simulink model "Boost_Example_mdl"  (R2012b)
settings: Solver=ode45  StartTime=0.0  StopTime=10.0  RelTol=1e-6
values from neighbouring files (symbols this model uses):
  Bg = ones(m,1)    [Boost_DC_M.m]    (also in Boost_DC_R100.m; Boost_Example.m; Boost_DC_Sliding.m)
  C = 200*microF    (= 0.0002)    [Boost_DC_M.m]    (also in Boost_DC_R100.m; Boost_Example.m; Boost_DC_Sliding.m)
  Im_0 = 0*(1:m)'    [Boost_DC_M.m]    (also in Boost_DC_R100.m; Boost_Example.m = In_Con(jj,1); Boost_DC_Sliding.m = In_Con(jj,1))
  Lm = diag(L1m(1:m))    [Boost_DC_M.m]    (also in Boost_DC_R100.m = eye(m)*L1; Boost_Example.m = eye(m)*L1; Boost_DC_Sliding.m = eye(m)*L1)
  R = 20*Ohm    (= 20)    [Boost_DC_M.m]    (also in Boost_DC_R100.m = 100; Boost_Example.m = 100; Boost_DC_Sliding.m = 100)
  Rm = diag(R1m(1:m))    [Boost_DC_M.m]    (also in Boost_DC_R100.m = eye(m)*R1; Boost_Example.m = eye(m)*R1; Boost_DC_Sliding.m = eye(m)*R1)
  Tc = Ts/50    (= 4e-07)    [Boost_DC_M.m]    (also in Boost_DC_R100.m; Boost_Example.m = 0.0002; Boost_DC_Sliding.m = 2e-05)
  Vc_0 = 0    [Boost_DC_M.m]    (also in Boost_DC_R100.m; Boost_Example.m = In_Con(jj,2); Boost_DC_Sliding.m = In_Con(jj,2))
  Vg = 100*Volt    (= 100)    [Boost_DC_M.m]    (also in Boost_DC_R100.m; Boost_Example.m; Boost_DC_Sliding.m)
undefined symbols (not defined in the file or in its folder): s1

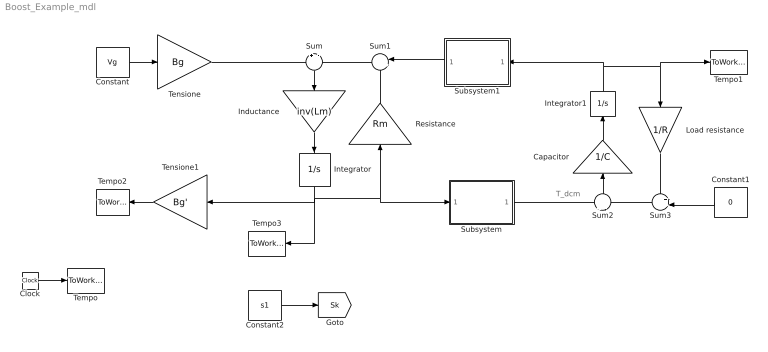
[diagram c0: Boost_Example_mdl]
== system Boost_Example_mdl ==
  note: T_dcm
  Capacitor : Gain  Gain=1/C
  Clock : Clock
  Constant : Constant  Value=Vg
  Constant1 : Constant  Value=0
  Constant2 : Constant  Value=s1
  Inductance : Gain  Gain=inv(Lm)  Multiplication=Matrix(K*u) (u vector)
  Integrator : Integrator  InitialCondition=Im_0  LimitOutput=on  LowerSaturationLimit=0
  Integrator1 : Integrator  InitialCondition=Vc_0
  Load resistance : Gain  Gain=1/R
  Resistance : Gain  Gain=Rm  Multiplication=Matrix(K*u) (u vector)
  Subsystem : Subsystem
  Subsystem1 : Subsystem
  Sum : Sum  Inputs=+|-
  Sum1 : Sum  Inputs=|++
  Sum2 : Sum  Inputs=+|-
  Sum3 : Sum  Inputs=++|
  Tempo : ToWorkspace  VariableName=t  SampleTime=Tc
  Tempo1 : ToWorkspace  VariableName=Vc  SampleTime=Tc
  Tempo2 : ToWorkspace  VariableName=Idc  SampleTime=Tc
  Tempo3 : ToWorkspace  VariableName=Im  SampleTime=Tc
  Tensione : Gain  Gain=Bg  Multiplication=Matrix(K*u) (u vector)
  Tensione1 : Gain  Gain=Bg'  Multiplication=Matrix(K*u) (u vector)
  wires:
  Clock/1 -> Tempo/1
  Sum/1 -> Inductance/1
  Inductance/1 -> Integrator/1
  Integrator/1 -> Resistance/1, Subsystem/1(In1), Tempo3/1, Tensione1/1
  Sum1/1 -> Sum/2
  Resistance/1 -> Sum1/2
  Subsystem/1(Out1) -> Sum2/1
  Sum2/1 -> Capacitor/1
  Capacitor/1 -> Integrator1/1
  Integrator1/1 -> Load resistance/1, Tempo1/1, Subsystem1/1(In1)
  Load resistance/1 -> Sum3/1
  Sum3/1 -> Sum2/2
  Constant1/1 -> Sum3/2
  Subsystem1/1(Out1) -> Sum1/1
  Constant/1 -> Tensione/1
  Tensione/1 -> Sum/1
  Tensione1/1 -> Tempo2/1
  Constant2/1 -> [Sk]

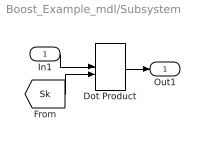
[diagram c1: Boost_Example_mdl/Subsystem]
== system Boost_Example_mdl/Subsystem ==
  In1 : Inport
  Dot Product : DotProduct
  Out1 : Outport
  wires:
  [Sk] -> Dot Product/2
  In1/1 -> Dot Product/1
  Dot Product/1 -> Out1/1

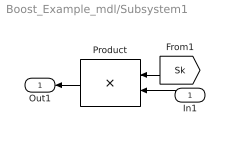
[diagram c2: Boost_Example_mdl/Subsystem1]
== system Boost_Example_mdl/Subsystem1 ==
  In1 : Inport
  Product : Product  Multiplication=Matrix(*)
  Out1 : Outport
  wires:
  [Sk] -> Product/1
  In1/1 -> Product/2
  Product/1 -> Out1/1
